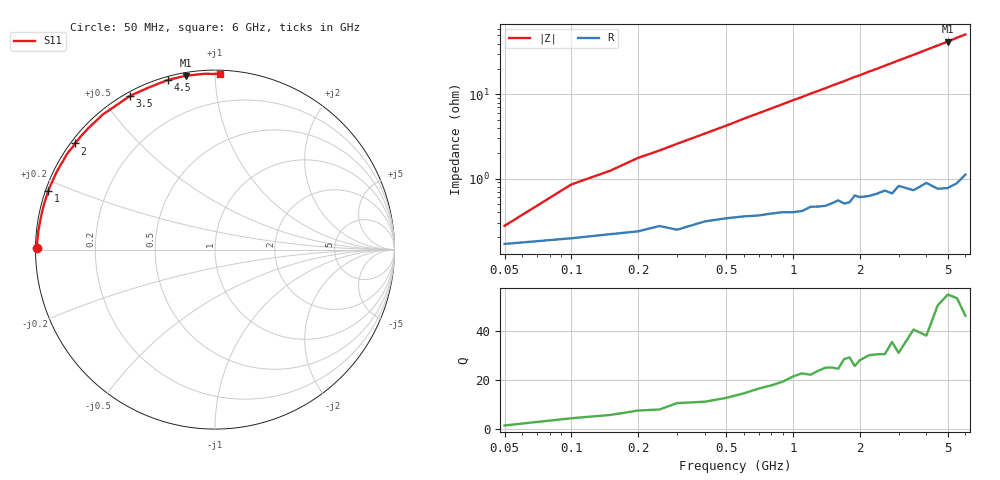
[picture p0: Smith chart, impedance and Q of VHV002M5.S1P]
! Infineon Technologies  Discrete & RF Semiconductors
! BB 814
! Si Tuning Diode in SOT23
! VR =
! S-Parameters:  July  1999
# GHz  S  MA  R  50
!  f  S11
! GHz  MAG  ANG
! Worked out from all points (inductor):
!   34 points, 50 MHz to 6 GHz, reference 50 ohm
!   read as one part to ground: L = 1.32 nH near 100 MHz
!   highest Q = 53.3 at 5 GHz (marker M1), where L = 1.34 nH
!   S11 on the Smith chart (normalised r, x): 50 MHz: 0.00, +0.00; 1 GHz: 0.01, +0.17; 2 GHz: 0.01, +0.34; 3.5 GHz: 0.01, +0.59; 4.5 GHz: 0.02, +0.76; 6 GHz: 0.02, +1.03
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0.05  0.9933 179.5
0.1  0.9922 178.1
0.15  0.9913 177.2
0.2  0.9906 176.0
0.3  0.9902 174.1
0.5  0.9867 170.3
0.6  0.986 168.3
0.8  0.985 164.5
1  0.9846 160.7
1.1  0.9842 158.9
1.4  0.9822 153.4
1.5  0.9811 151.5
1.6  0.9796 149.8
1.7  0.9815 148.0
1.8  0.981 146.2
1.9  0.9774 144.3
2  0.9786 142.8
2.2  0.9784 139.2
2.4  0.9774 136.1
2.6  0.9761 132.6
2.8  0.9784 129.6
3  0.9743 126.3
3.5  0.9786 119.0
4  0.9759 111.9
4.5  0.981 105.4
5  0.9821 99.6
5.5  0.9814 93.4
6  0.9785 88.4
